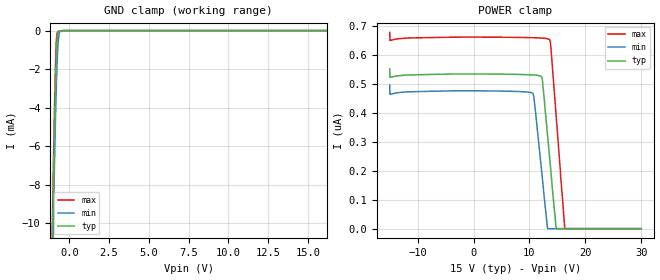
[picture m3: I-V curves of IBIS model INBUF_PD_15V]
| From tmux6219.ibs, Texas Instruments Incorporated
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| Model3
[Model]   INBUF_PD_15V
Model_type   Input
Vinl = 0.8
Vinh = 1.3
|   typ   min   max
C_comp   1.85pF   1.7pF   2.1pF
[Voltage Range]   15   13.5   16.5
[Temperature Range]   27   130   -40
[Power Clamp Reference]   15   13.5   16.5
[GND Clamp Reference]   0   0   0
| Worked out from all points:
|   GND clamp passes 1 mA (typ) near -0.80 V on its own axis
[GND Clamp]
|   Voltage   I(typ)   I(min)   I(max)
-15V      -759mA     -758.2mA   -760mA
-1.095V   -12.42mA   -14mA      -11.35mA
-1.05V    -10.29mA   -11.93mA   -9.178mA
-1.005V   -8.227mA   -9.918mA   -7.071mA
-915mV    -4.411mA   -6.162mA   -3.214mA
-870mV    -2.785mA   -4.496mA   -1.662mA
-825mV    -1.491mA   -3.048mA   -614uA
-780mV    -631uA     -1.881mA   -163.9uA
-735mV    -199.9uA   -1.026mA   -65.16uA
-645mV    -28.51uA   -175.5uA   -35.22uA
-330mV    -148.9nA   -479.8nA   -157.8nA
30V       0A         0A         0A
[POWER Clamp]
|   Voltage   I(typ)   I(min)   I(max)
-15V      553nA      496.7nA    678.9nA
-14.96V   522.9nA    464.5nA    650.7nA
-3.75V    534.9nA    476.7nA    662.4nA
10.65V    531.8nA    466.8nA    660.5nA
10.96V    531.4nA    426.8nA    660.3nA
12.27V    520.8nA    183.2nA    659.3nA
13.21V    329.5nA    4.066nA    656.9nA
13.62V    244.6nA    0A         654.3nA
13.8V     206.8nA    0A         637.5nA
14.74V    7.393nA    0A         400.5nA
16.32V    0A         0A         1.378nA
30V       0A         0A         0A
